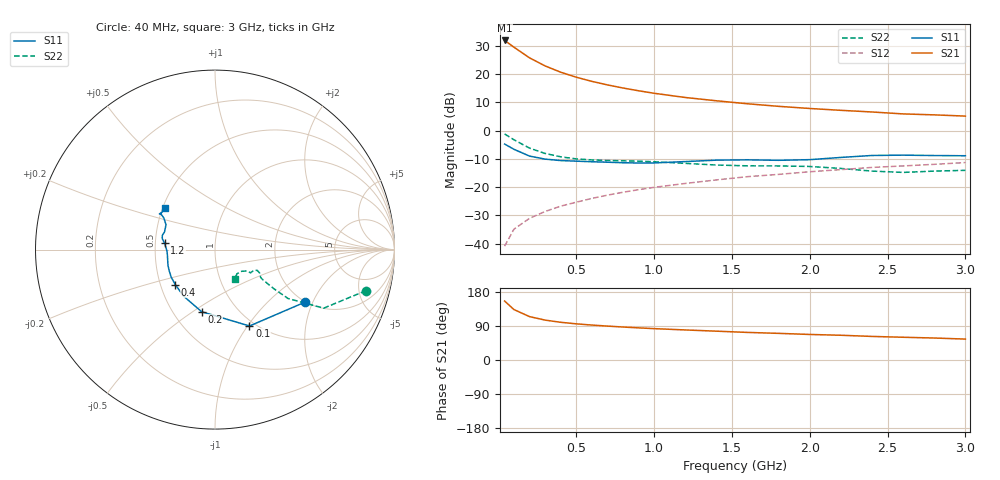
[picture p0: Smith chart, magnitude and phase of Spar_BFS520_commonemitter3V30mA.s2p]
! Filename:  BFS520F.S2P  Version:  4.0
! NXP part #: BFS520  Date: Jun 1994
! Bias condition: Vce=3V, Ic=30mA
#  MHz  S  MA  R  50
! Freq  S11  S21  S12  S22  !GUM [dB]
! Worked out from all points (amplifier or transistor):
!   21 points, 40 MHz to 3 GHz, reference 50 ohm
!   highest |S21| = 31.9 dB at 40 MHz (marker M1)
!   |S21| within 3 dB of that: start of sweep to 116.3 MHz
!   unconditionally stable (mu >= 1): 470.3 MHz to end of sweep
!   at 300 MHz: K = 0.89, MSG = 25.8 dB, |S12| = -28.6 dB
!   at 1 GHz: K = 1.09, MAG = 14.8 dB, |S12| = -20.1 dB
!   at 3 GHz: K = 1.04, MAG = 6.9 dB, |S12| = -11.3 dB
!   S11 on the Smith chart (normalised r, x): 40 MHz: 1.97, -1.74; 100 MHz: 0.94, -1.02; 200 MHz: 0.69, -0.54; 400 MHz: 0.60, -0.26; 1.2 GHz: 0.56, +0.04; 3 GHz: 0.52, +0.27
40  0.579 -30.5  39.47 155.6  0.009 77.8  0.872 -15.2
100  0.467 -65.7  29.99 133.1  0.018 67.5  0.688 -28.3
200  0.354 -102.1  19.42 114.5  0.028 64.7  0.49 -33.8
300  0.313 -123.9  13.98 105.3  0.037 66.9  0.394 -33.6
400  0.295 -138.6  10.82 99.5  0.046 69.1  0.344 -32.8
500  0.288 -148.1  8.827 95.4  0.054 70.9  0.316 -32.2
600  0.281 -155.4  7.452 92.2  0.063 72.1  0.303 -31.7
700  0.276 -161.7  6.453 89.5  0.072 73.1  0.296 -31.1
800  0.27 -167.5  5.684 87.0  0.081 73.8  0.292 -30.1
900  0.267 -173.2  5.079 84.8  0.09 74.1  0.288 -28.9
1000  0.268 -178.7  4.585 82.8  0.099 74.5  0.281 -27.7
1200  0.283 172.9  3.861 79.3  0.116 74.7  0.263 -26.2
1400  0.3 168.3  3.375 76.1  0.134 75.2  0.246 -27.9
1600  0.304 165.0  2.987 72.8  0.153 74.4  0.238 -32.0
1800  0.298 160.5  2.691 70.3  0.168 74.3  0.237 -33.4
2000  0.306 153.1  2.466 67.4  0.187 73.7  0.232 -33.3
2200  0.335 148.3  2.287 65.3  0.204 73.7  0.214 -33.8
2400  0.363 146.5  2.138 62.2  0.223 73.0  0.192 -38.9
2600  0.368 147.3  1.976 60.0  0.237 71.9  0.182 -47.8
2800  0.362 145.3  1.9 58.0  0.253 71.8  0.192 -53.9
3000  0.359 140.3  1.808 55.2  0.272 71.0  0.198 -55.8
